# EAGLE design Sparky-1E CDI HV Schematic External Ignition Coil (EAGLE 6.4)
Miniature low power CDi for RC and other small battery powered engines.
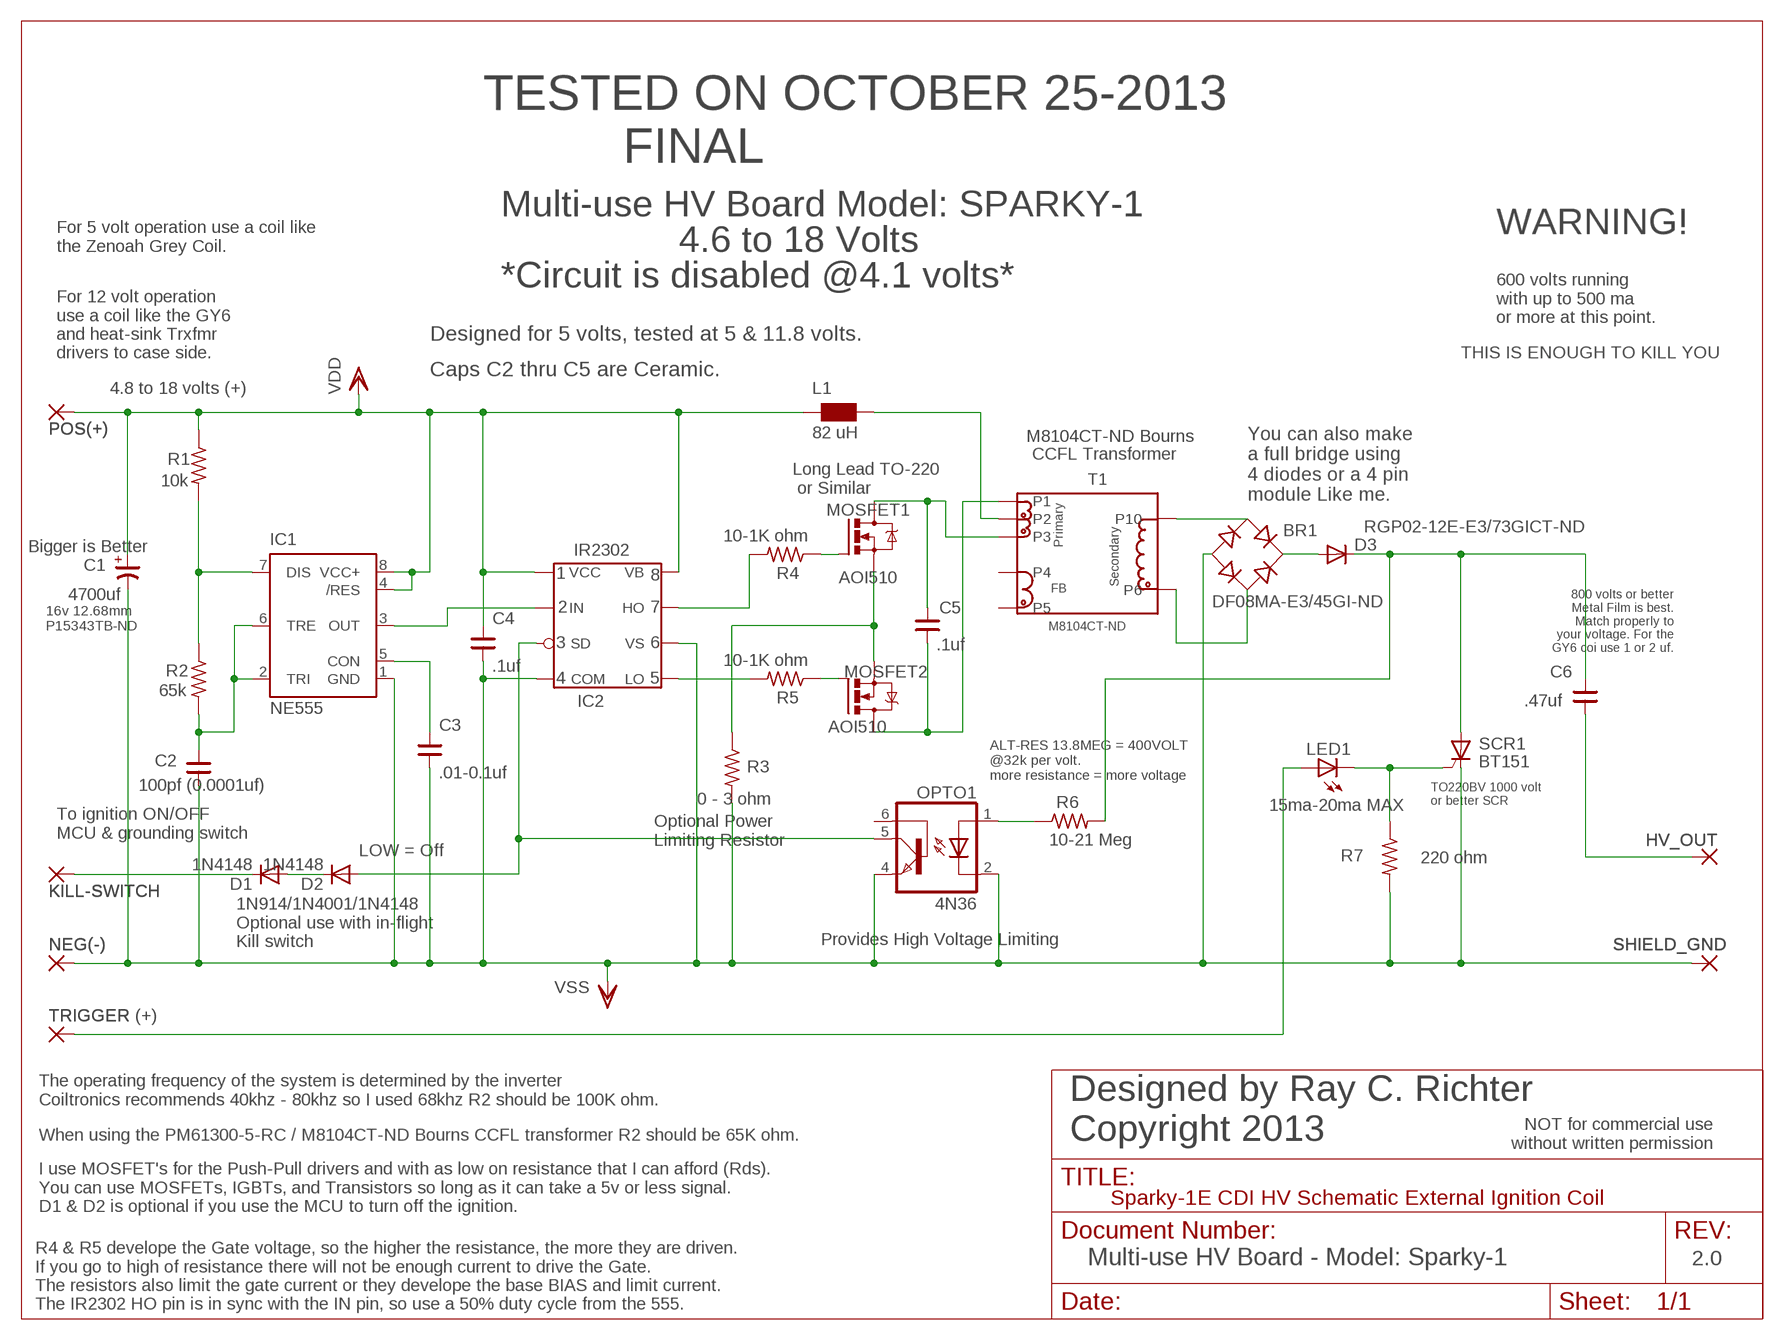
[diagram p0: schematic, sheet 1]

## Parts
BR1  DF08MA-E3/45GI-ND  B-DIL  [B-DIL]
C1  4700uf  CP-E-075X160  [E-075X160]
C2  100pf (0.0001uf)  CNP-C050-075X030  [C050-075X030]
C3  .01-0.1uf  CNP-C050-075X030  [C050-075X030]
C4  .1uf  CNP-C050-075X030  [C050-075X030]
C5  .1uf  CNP-C050-075X030  [C050-075X030]
C6  .47uf  CNP-C275-320X100  [C275-320X100]
D1  1N4148  [RAD2,5L]
D2  1N4148  [RAD2,5L]
D3  RGP02-12E-E3/73GICT-ND  DIODE-C1702-05  [C1702-05]
HV_OUT  HV_OUT  3,81/1,1  [3,81/1,1]
IC1  NE555  [DIL-08]
IC2  IR2302  [DIL8]
KILL-SWITCH  KILL-SWITCH  2,54/0,8  [2,54/0,8]
L1  82 uH  WE-TI_L  [WE-TI_L]
LED1  15ma-20ma MAX  LED5MM  [LED5MM]
MOSFET1  AOI510  IRF520  [TO220BV]
MOSFET2  AOI510  IRF520  [TO220BV]
NEG(-)  NEG(-)  2,54/0,8  [2,54/0,8]
OPTO1  4N36  4N37M  [DIL06]
POS(+)  POS(+)  2,54/0,8  [2,54/0,8]
R1  10k  R-US_0207/2V  [0207/2V]
R2  65k  R-US_0207/2V  [0207/2V]
R3  0 - 3 ohm  R-US_0204/7  [0204/7]
R4  10-1K ohm  R-US_0207/2V  [0207/2V]
R5  10-1K ohm  R-US_0204/7  [0204/7]
R6  10-21 Meg  R-US_0207/2V  [0207/2V]
R7  220 ohm  R-US_0204/7  [0204/7]
SCR1  BT151  BT151TO220BV  [TO220BV]
SHIELD_GND  SHIELD_GND  3,81/1,1  [3,81/1,1]
T1  M8104CT-ND  CCFL-INVERTERCCFL-INVERTER-SMD  [CCFL-INVERTER_SMD]
TRIGGER  TRIGGER (+)  2,54/0,8  [2,54/0,8]

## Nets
N$2: LED1.A TRIGGER.1(P)
N$3: C6.2 D3.C R6.2 SCR1.A
N$4: BR1.AC2 T1.P$6(P6)
N$5: C5.2 MOSFET1.D T1.P$3(P3)
N$6: BR1.+ D3.A
N$7: MOSFET2.G R5.1
N$8: MOSFET1.G R4.1
N$9: IC2.P$5(LO) R5.2
N$10: IC2.P$7(HO) R4.2
N$11: BR1.AC1 T1.P$10(P10)
N$12: LED1.K(C) R7.1 SCR1.G
N$14: OPTO1.1(A) R6.1
N$15: IC1.3(OUT) IC2.P$2(IN)
N$16: D2.A IC2.P$3(SD) OPTO1.5(COL)
N$18: C5.1 MOSFET2.D T1.P$1(P1)
N$19: C3.2 IC1.5(CON)
N$21: C6.1 HV_OUT.1(P)
N$22: C2.2 IC1.2(TRI) IC1.6(TRE) R2.2
N$23: D1.C KILL-SWITCH.1(P)
N$24: IC1.7(DIS) R1.2 R2.1
N$25: D1.A D2.C
N$26: MOSFET1.S MOSFET2.S R3.1
VDD: C1.+ C4.2 IC1.4(/RES) IC1.8(VCC+) IC2.P$1(VCC) IC2.P$8(VB) L1.1 L1.2 POS(+).1(P) R1.1 T1.P$2(P2)
VSS: BR1.- C1.- C2.1 C3.1 C4.1 IC1.1(GND) IC2.P$4(COM) IC2.P$6(VS) NEG(-).1(P) OPTO1.2(C) OPTO1.4(EMI) R3.2 R7.2 SCR1.K SHIELD_GND.1(P)
Unconnected: OPTO1.6(BAS) T1.P$4(P4) T1.P$5(P5)

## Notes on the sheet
- TESTED ON OCTOBER 25-2013
            FINAL
- Multi-use HV Board Model: SPARKY-1
- WARNING!
- For 5 volt operation use a coil like
  the Zenoah Grey Coil.
- 4.6 to 18 Volts
- *Circuit is disabled @4.1 volts*
- 600 volts running
  with up to 500 ma 
  or more at this point.
- Designed for 5 volts, tested at 5 & 11.8 volts.
- For 12 volt operation
  use a coil like the GY6
  and heat-sink Trxfmr
  drivers to case side.
- THIS IS ENOUGH TO KILL YOU
- Caps C2 thru C5 are Ceramic.
- 4.8 to 18 volts (+)
- M8104CT-ND Bourns
- CCFL Transformer
- Long Lead TO-220
   or Similar
- You can also make
  a full bridge using
  4 diodes or a 4 pin
  module Like me.
- Bigger is Better
- 800 volts or better
  Metal Film is best.
  Match properly to
  your voltage. For the
  GY6 coi use 1 or 2 uf.
- 16v 12.68mm
  P15343TB-ND
- ALT-RES 13.8MEG = 400VOLT
  @32k per volt. 
  more resistance = more voltage
- TO220BV 1000 volt
  or better SCR
- To ignition ON/OFF
  MCU & grounding switch
- Optional Power
  Limiting Resistor
- LOW = Off
- Provides High Voltage Limiting
- 1N914/1N4001/1N4148
  Optional use with in-flight
  Kill switch
- The operating frequency of the system is determined by the inverter
  Coiltronics recommends 40khz - 80khz so I used 68khz R2 should be 100K ohm.
- NOT for commercial use
  without written permission
- When using the PM61300-5-RC / M8104CT-ND Bourns CCFL transformer R2 should be 65K ohm.
- Designed by Ray C. Richter
  Copyright 2013
- I use MOSFET's for the Push-Pull drivers and with as low on resistance that I can afford (Rds).
  You can use MOSFETs, IGBTs, and Transistors so long as it can take a 5v or less signal.
  D1 & D2 is optional if you use the MCU to turn off the ignition.
- Multi-use HV Board - Model: Sparky-1 | 2.0
- R4 & R5 develope the Gate voltage, so the higher the resistance, the more they are driven.
  If you go to high of resistance there will not be enough current to drive the Gate.
  The resistors also limit the gate current or they develope the base BIAS and limit current.
  The IR2302 HO pin is in sync with the IN pin, so use a 50% duty cycle from the 555.

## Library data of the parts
BR1 = rectifier:B-DIL: RECTIFIER
C1 = cap-master:CP-: POLARIZED CAP
C2-C6 = cap-master:CNP-: NON-POLARIZED CAP
D1 D2 = diode:1N4148: DIODE
D3 = diode:DIODE-: DIODE
HV_OUT SHIELD_GND = wirepad:3,81/1,1: THROUGH-HOLE PAD
IC1 = st-microelectronics:NE555: General purpose bipolar Timer; MF: Arrow Electronics; MPN: NE555N; OC_FARNELL: 1467742; OC_NEWARK: 89K1486
IC2 = MY-Custom:IR2302
KILL-SWITCH NEG(-) POS(+) TRIGGER = wirepad:2,54/0,8: THROUGH-HOLE PAD
L1 = wuerth-elektronik:WE-TI: Radial Leaded Wire Wound Inductor WE-TI
LED1 = led:LED: LED
MOSFET1 MOSFET2 = transistor-power:IRF520: HEXFET Power MOSFET
OPTO1 = optocoupler:4N*?M: General Purpose 6-Pin Phototransistor Optocouplers Source: http://www.fairchildsemi.com/ds/4N/4N35-M.pdf; MPN: 4N37-M; OC_FARNELL: 1021353; OC_NEWARK: 98K9125
R1-R7 = R-C-L-E:R-US_: RESISTOR, American symbol
SCR1 = triac:BT151: THYRISTOR
T1 = MY_STUFF:CCFL-INVERTER; MANUFACTURER: Cooper Bussmann

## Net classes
0 default: clearance 0.355 mm

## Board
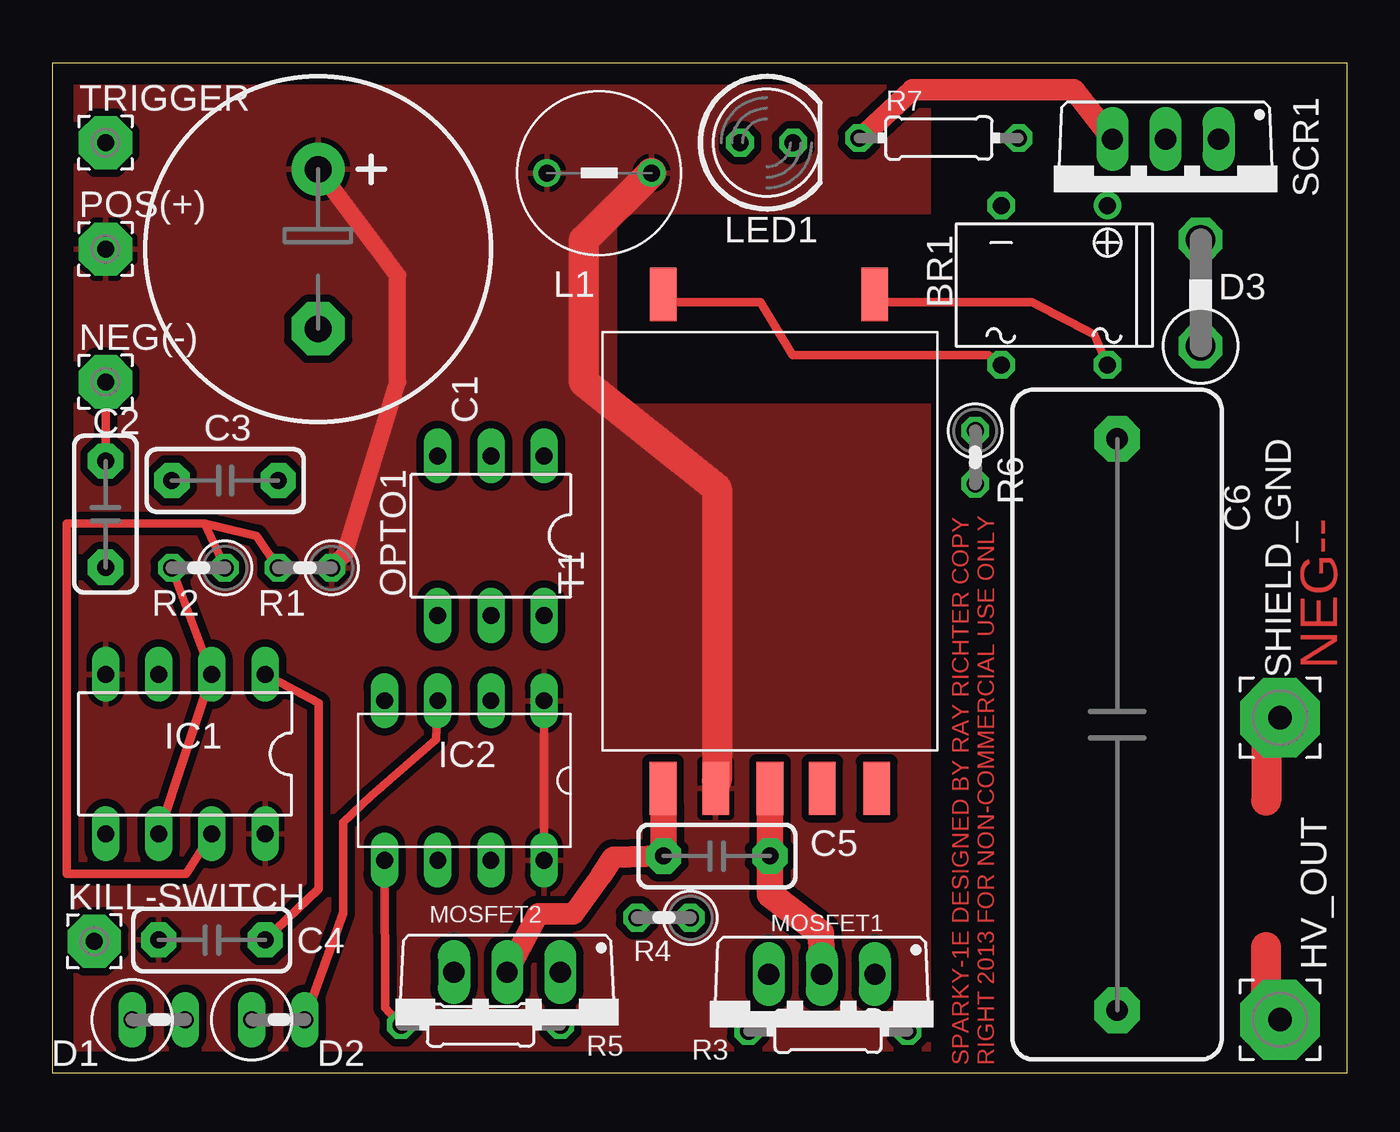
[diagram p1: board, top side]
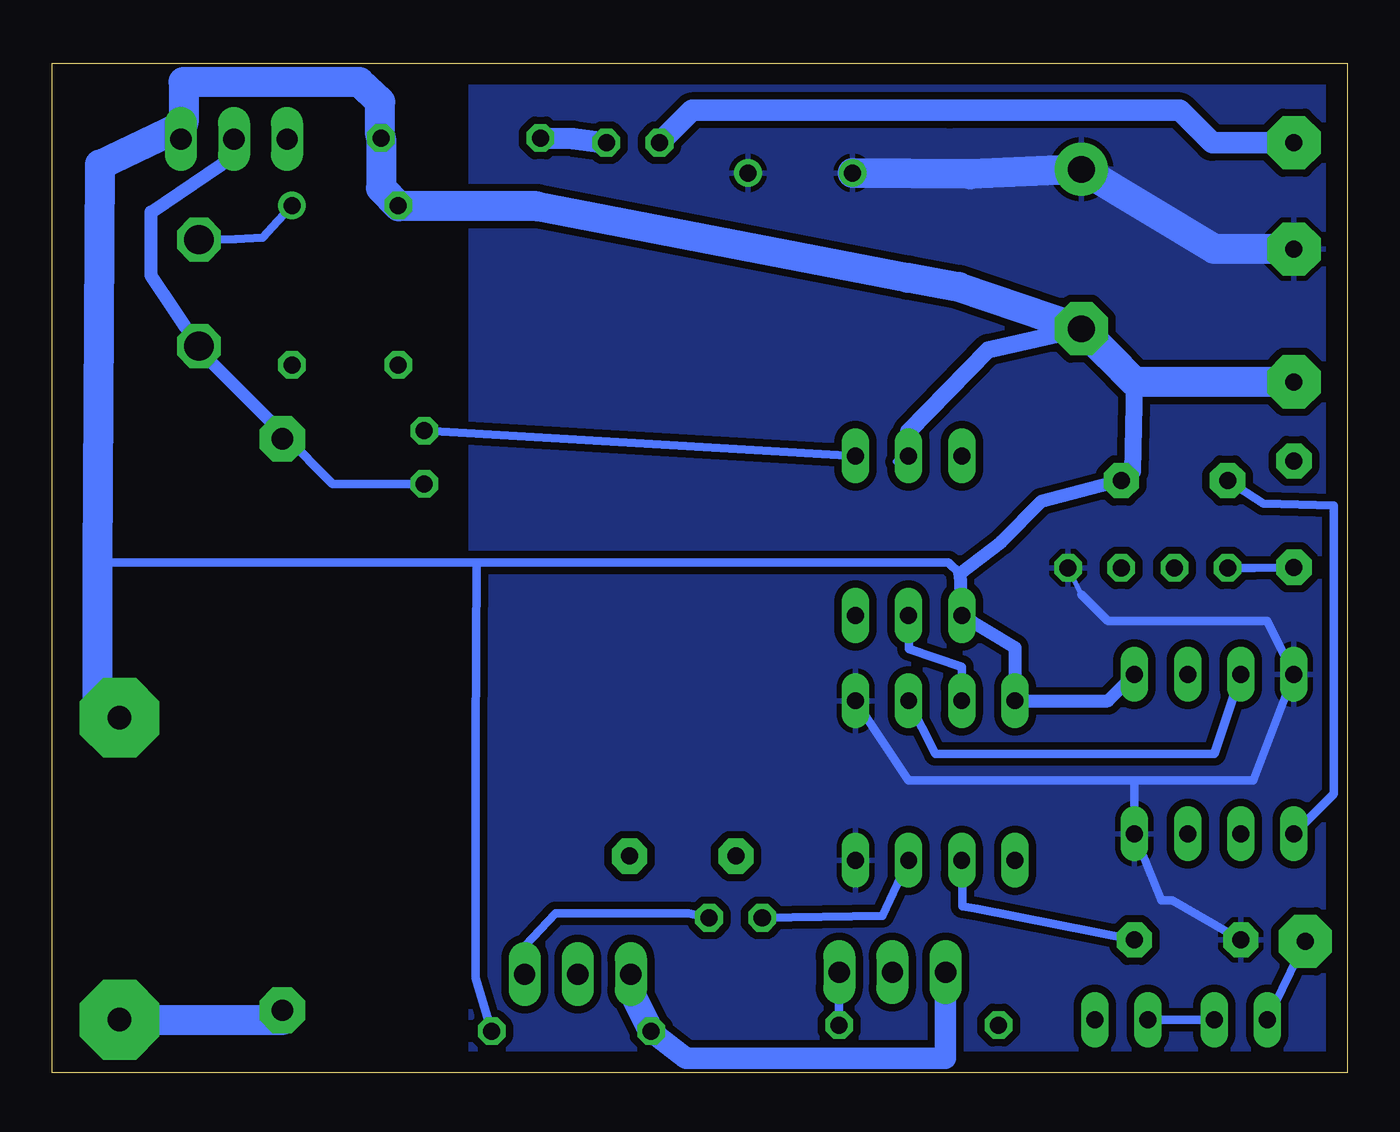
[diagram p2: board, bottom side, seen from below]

Size 61.87 x 48.25 mm. Coordinates in mm from the lower left corner, seen from the top.
Outline: 0,0 61.87,0 61.87,48.25 0,48.25 0,0
Copper layers (1*16): Top 0.035mm / dielectric 1.5mm / Bottom 0.035mm
Design rules "Sparky-1 CDI HV Schematic IR2302-NE555": minimum track width 10mil, minimum drill 24mil, track to track 0.355mm, track to pad 0.355mm, pad to pad 0.355mm, via to via 0.355mm, smd to smd 8mil, copper to edge 40mil, drill to drill 8mil, minimum pad ring 10mil, minimum via ring 8mil, stop-mask expansion 4mil, vias tented up to drill 0mil, thermal gap 10mil
tRestrict: area 42,0 to 62,48; area 27,32 to 42,41
bRestrict: area 42,0 to 62,48

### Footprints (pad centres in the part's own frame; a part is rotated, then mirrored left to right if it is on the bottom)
B-DIL = drill 0.813: + -2.54,-3.81 | drill 0.813 octagon: - 2.54,-3.81; AC1 2.54,3.81; AC2 -2.54,3.81
E-075X160 = drill 1.27 pad 2.54: + -3.81,0 | drill 1.27 pad 2.54 octagon: - 3.81,0
C050-075X030 = drill 0.813 pad 1.676 octagon: 1 -2.54,0; 2 2.54,0
C275-320X100 = drill 1.016 pad 2.184 octagon: 1 -13.652,0; 2 13.652,0
RAD2,5L = drill 0.813 long: A 1.27,0; C -1.27,0
C1702-05 = drill 1.397 octagon: A 2.54,0; C -2.54,0
3,81/1,1 = drill 1.118 pad 3.81 octagon: 1 0,0
DIL-08 = drill 0.813 long: 1 -3.81,-3.81; 2 -1.27,-3.81; 3 1.27,-3.81; 4 3.81,-3.81; 5 3.81,3.81; 6 1.27,3.81; 7 -1.27,3.81; 8 -3.81,3.81
DIL8 = drill 0.8 long: P$1 -3.81,3.81; P$2 -3.81,1.27; P$3 -3.81,-1.27; P$4 -3.81,-3.81; P$5 3.81,-3.81; P$6 3.81,-1.27; P$7 3.81,1.27; P$8 3.81,3.81
2,54/0,8 = drill 0.813 pad 2.54 octagon: 1 0,0
WE-TI_L = drill 0.813: 1 -2.5,0; 2 2.5,0
LED5MM = drill 0.813 octagon: A -1.27,0; K 1.27,0
TO220BV = drill 1.016 long: D 0,-2.54; G -2.54,-2.54; S 2.54,-2.54
DIL06 = drill 0.813 long: 1 -2.54,-3.81; 2 0,-3.81; 3 2.54,-3.81; 4 2.54,3.81; 5 0,3.81; 6 -2.54,3.81
0207/2V = drill 0.813 octagon: 1 -1.27,0; 2 1.27,0
0204/7 = drill 0.813 octagon: 1 -3.81,0; 2 3.81,0
TO220BV' = drill 1.016 long: A 0,-2.54; G 2.54,-2.54; K -2.54,-2.54
CCFL-INVERTER_SMD = smd 2.54 x 1.27: P$1 -11.8,5.11; P$2 -11.8,2.6; P$3 -11.8,0; P$4 -11.8,-2.5; P$5 -11.8,-5.1; P$6 11.8,-5; P$10 11.8,5.1

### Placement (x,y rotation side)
BR1  47.88,37.64 180 top
C1  12.7,39.37 270 top
C2  2.54,26.7 270 top
C3  8.26,28.3 180 top
C4  7.62,6.35 180 top
C5  31.75,10.36 0 top
C6  50.88,16.64 90 top
D1  5.08,2.54 0 top
D2  10.79,2.54 0 top
D3  54.87,37.27 90 top
HV_OUT  58.66,2.54 0 top
IC1  6.35,15.24 180 top
IC2  19.68,13.97 270 top
KILL-SWITCH  2,6.29 0 top
L1  26.13,43 180 top
LED1  34.13,44.45 0 top
MOSFET1  36.77,2.17 180 top
MOSFET2  21.73,2.27 180 top
NEG(-)  2.54,33.02 0 top
OPTO1  20.95,25.67 180 top
POS(+)  2.54,39.37 0 top
R1  12.06,24.13 180 top
R2  6.99,24.13 180 top
R3  37.06,2 0 top
R4  29.22,7.41 180 top
R5  20.46,2.29 180 top
R6  44.1,29.41 270 top
R7  42.36,44.67 0 top
SCR1  BT151  [TO220BV']  53.19,42.08 180 top
SHIELD_GND  58.66,16.97 0 top
T1  34.29,25.4 90 top
TRIGGER  2.54,44.45 0 top

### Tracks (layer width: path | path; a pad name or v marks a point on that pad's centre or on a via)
N$1
  Top 1.422: 59,17 58,17 58,13
N$2
  Bottom 1.016: TRIGGER.1 6.45,44.45 8,46 19,46 31.31,46 LED1.A
N$3
  Bottom 0.254: 54.91,34.76 D3.C | 50.8,30.48 C6.2
  Bottom 0.406: 53.14,43.85 53.14,43.82 | 50.8,30.48 48.47,28.14 R6.2
  Bottom 0.61: 53.14,43.85 57.15,41.14 57.15,38.1 54.91,34.76 | 53.14,43.82 SCR1.A | 50.8,30.48 54.61,34.29 D3.C
N$4
  Top 0.254: 39.37,36.83 T1.P$6
  Top 0.406: 39.37,36.83 46.8,36.83 49.8,35.29 BR1.AC2
N$5
  Top 0.254: 34.29,10.16 C5.2 | 34.29,12.7 T1.P$3 | 34.29,10.16 C5.2 | 34.29,10.16 C5.2
  Top 1.27: C5.2 34.29,12.7 | 34.29,10.16 34.29,8.52 36.73,6.68 MOSFET1.D
N$6
  Bottom 0.406: BR1.+ 51.1,40.71 51.81,39.91 53.11,39.84 D3.A
N$7
  Bottom 0.406: MOSFET2.G R5.1
N$8
  Bottom 0.406: R4.1 31.48,7.62 37.83,7.62 39.27,6.08 MOSFET1.G
N$9
  Top 0.406: IC2.P$5 15.9,3.1 R5.2
N$10
  Bottom 0.406: IC2.P$7 22.2,7.5 R4.2
N$11
  Top 0.254: 29.21,36.83 T1.P$10
  Top 0.406: 29.21,36.83 33.83,36.83 35.37,34.29 40.64,34.29 44.72,34.29 BR1.AC1
N$12
  Top 1.016: 38.6,44.65 41.1,46.99 48.8,46.99 SCR1.G
  Top 1.27: 38.6,44.65 R7.1
  Bottom 0.254: 35.56,44.45 LED1.K | 37,44.65 R7.1
  Bottom 1.016: 35.56,44.45 37,44.65 R7.1
N$13
  Bottom 1.27: 55.6,45.4 55.7,45.3
  Bottom 1.422: 46.2,44.8 46.2,46.4 47.2,47.35 55.6,47.35 55.6,45.4
N$14
  Bottom 0.406: OPTO1.1 R6.1
N$15
  Bottom 0.406: IC2.P$2 19.68,15.24 6.35,15.24 IC1.3
N$16
  Top 0.406: IC2.P$3 18.34,15.94 15.24,13.24 13.9,11.97 13.9,7.62 D2.A
  Bottom 0.406: OPTO1.5 20.95,20.25 18.4,19.4 IC2.P$3
N$17
  Top 1.422: 59,3 58,3 58,6
N$18
  Top 0.254: 29.21,12.7 T1.P$1 | 29.21,10.16 C5.1
  Top 1.016: MOSFET2.D 23.2,7.6 24.9,7.6 26.2,9.4 26.8,10.3 C5.1
  Top 1.27: C5.1 29.21,12.7
N$19
  Bottom 0.406: C3.2 4.01,27.2 0.64,27.1 0.64,13.34 IC1.5
N$21
  Bottom 0.61: 50.8,2.54 C6.1 | 58.42,2.54 HV_OUT.1
  Bottom 1.422: 58.42,2.54 50.8,2.54
N$22
  Top 0.406: IC1.6 6.35,15.24 IC1.2 R2.2
  Bottom 0.406: C2.2 4.45,24.13 R2.2
N$23
  Bottom 0.406: KILL-SWITCH.1 D1.C
N$24
  Top 0.254: 7.29,26.26 R2.1
  Top 0.406: IC1.7 6.4,9.5 0.7,9.5 0.69,26.24 7.29,26.26 | 7.29,26.26 9.76,25.66 R1.2 | 7.29,26.26 R2.1
N$25
  Bottom 0.406: D2.C 7.08,2.54 D1.A
N$26
  Bottom 0.254: 34.19,3.91 34.12,3.74
  Bottom 1.016: MOSFET2.S 19.2,0.7 31.6,0.7 R3.1
  Bottom 1.27: 34.12,3.74 R3.1 | 34.19,3.91 MOSFET1.S
VDD
  Top 0.254: 31.75,13.97 T1.P$2
  Top 0.406: IC2.P$1 IC2.P$8
  Top 0.813: C1.+ 15.44,39.52 16.51,38.1 16.51,33.02 13.97,24.77 R1.1
  Top 1.422: 31.75,13.97 31.75,27.94 25.4,33.02 25.4,39.8 L1.1
  Bottom 0.254: 12.7,22.86 R1.1
  Bottom 0.406: 12.7,22.86 11.43,21.59 3.81,21.59 IC1.4 4.48,13.97 10.16,13.97 | IC2.P$1 20.95,13.97 10.16,13.97 | 10.16,13.97 IC1.8 8.89,8.26 8.35,8.26 C4.2
  Bottom 1.422: POS(+).1 6.35,39.37 C1.+ 18.02,42.94 L1.2
  pour Bottom: 0,48 62,48 62,0 0,0
  pour Top: 0,48 62,48 62,0 0,0
VSS
  Top 0.406: NEG(-).1 C2.1 | C4.1 12.73,8.79 12.73,17.68 IC1.1
  Bottom 0.254: 21.59,29.21 21.1,29.21 | 21.59,29.21 21.1,29.21 | 21.59,29.21 21.1,29.21 | 21.59,29.21 21.1,29.21 | 21.59,29.21 21.1,29.21 | 21.59,29.21 21.1,29.21 | 21.59,29.21 21.1,29.21 | 21.59,29.21 21.1,29.21 | 20.59,30.48 21.1,30.42 | 20.59,30.48 21.1,30.42 | 21.59,29.21 21.1,29.21 | 21.59,29.21 21.1,29.21 | 20.59,30.48 21.1,30.42 | 20.59,30.48 21.1,30.42 | 20.59,30.48 21.1,30.42 | 21.59,29.21 OPTO1.2 21.59,29.21 | 21.59,29.21 20.59,30.48
  Bottom 0.406: 41.6,24.4 59.69,24.4 | C4.1 17.68,7.85 18.38,7.96 IC2.P$6 | R3.2 41.64,4.54 41.64,15.78 41.6,24.4 | 41.6,24.4 19.05,24.4 18.51,23.86
  Bottom 0.61: IC1.1 11.43,17.78 IC2.P$4 15.88,20.32 OPTO1.4 18.51,23.86 16.51,25.4 14.61,27.3 C3.1 | 55.78,45.22 SCR1.K
  Bottom 0.813: 10.16,33.02 10.26,28.74 C3.1 | OPTO1.2 20.95,30.66 17.14,34.56 C1.-
  Bottom 1.016: 59.69,17.78 SHIELD_GND.1 | 45.32,41.41 BR1.-
  Bottom 1.422: NEG(-).1 10.16,33.02 11.43,34.29 C1.- 18.56,37.56 21,38 38.7,41.41 45.32,41.41 | R7.2 46.17,42.28 BR1.- | 55.78,45.22 59.59,43.41 59.69,24.4 59.69,17.78

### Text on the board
Top: NEG-- | SPARKY-1E DESIGNED BY RAY RICHTER COPY / RIGHT 2013 FOR NON-COMMERCIAL USE ONLY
